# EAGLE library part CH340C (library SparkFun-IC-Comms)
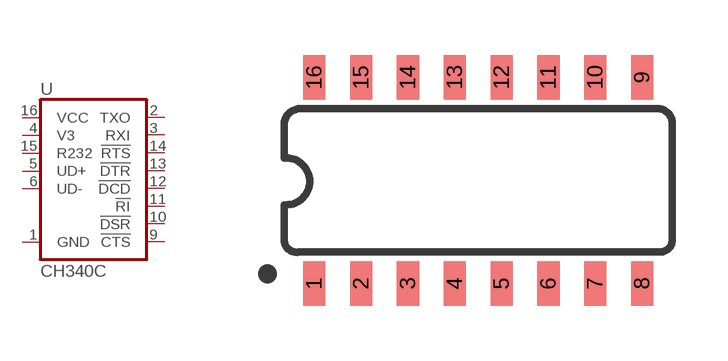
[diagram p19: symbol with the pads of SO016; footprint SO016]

Designator prefix U

## CH340C (PROD_ID: IC-14038)  [SO016]
1  GND
2  TXO
3  RXI
4  V3
5  UD+
6  UD-
9  !CTS
10  !DSR
11  !RI
12  !DCD
13  !DTR
14  !RTS
15  R232
16  VCC

## Footprint SO016 (pad centres in mm)
smd 0.6 x 1.2: 1 -4.445,-2.8; 2 -3.175,-2.8; 3 -1.905,-2.8; 4 -0.635,-2.8; 5 0.635,-2.8; 6 1.905,-2.8; 7 3.175,-2.8; 8 4.445,-2.8; 9 4.445,2.8; 10 3.175,2.8; 11 1.905,2.8; 12 0.635,2.8; 13 -0.635,2.8; 14 -1.905,2.8; 15 -3.175,2.8; 16 -4.445,2.8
